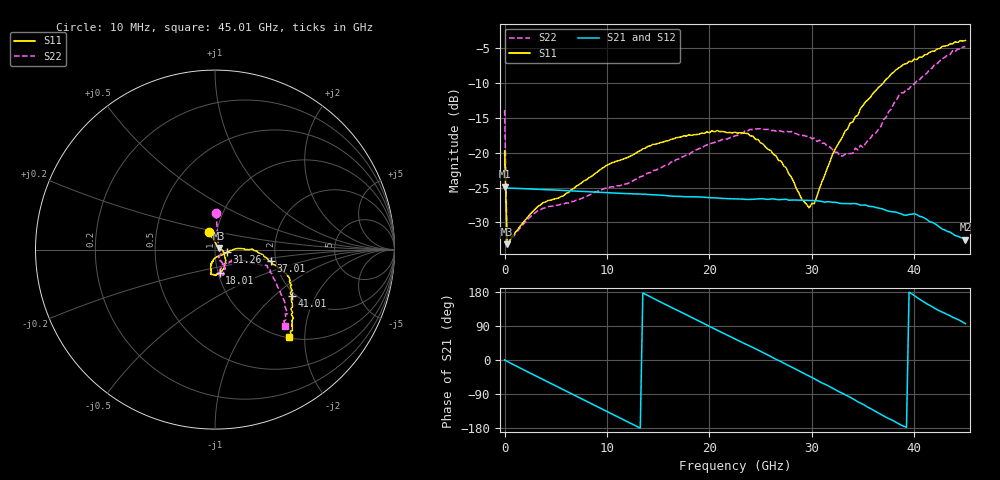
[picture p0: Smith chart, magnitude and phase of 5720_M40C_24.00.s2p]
! Device:  ADRF5720
! Description: 0.5dB LSB GaAs MMIC 6-bit Digital Attenuator
! Frequency:  0.000009 -  40 GHz
! Ports:
!	RF1	= Port 1
!	RF2	= Port 2
! Vdd:  3.3 Volt
! Vss:  -3.3 Volt
! Control:  0/3.3 Volt
! State:  24.00 dB attenuation
! Data:  The device was measured using G-S-G Probes on a matrix board.
!  Data was collected using an calibrated 4 port network analyzer.
!  The reference plane for this measurement is at the launchers.
! Note:  Analog Devices supplies this data as a sample of measured data
!  for this product.  Your particular data for this product may vary.
!  Data was taken at -40 degrees C.
!  Analog Devices reserves the right to change this data at anytime.
# GHZ S DB R 45.0
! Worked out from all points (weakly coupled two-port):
!   181 points, 10 MHz to 45.01 GHz, reference 45 ohm
!   highest |S21| = -24.90 dB at 10 MHz (marker M1); lowest = -32.5 dB at 45.01 GHz (marker M2)
!   lowest |S11| = -33.2 dB at 260 MHz (marker M3), VSWR 1.04, Z = 46.8 + j0.913 ohm
!   |S11| at or under -10 dB: start of sweep to 36.98 GHz
!   |S22| runs from -33.4 to -4.8 dB; largest |S21 - S12| = 0.00021
!   S11 on the Smith chart (normalised r, x): 10 MHz: 0.92, +0.18; 18.01 GHz: 1.02, -0.27; 31.26 GHz: 1.14, -0.03; 37.01 GHz: 1.88, -0.27; 41.01 GHz: 1.91, -1.33; 45.01 GHz: 1.02, -1.67
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0.01  -19.75 109.5  -24.90 0.3  -24.91 0.3  -13.88 88.3
0.26  -33.18 26.4  -25.08 -3.7  -25.10 -3.8  -33.42 22.4
3.26  -27.71 -4.6  -25.26 -44.8  -25.28 -44.8  -28.31 -29.3
7.76  -24.05 -32.4  -25.57 -105.5  -25.59 -105.5  -26.41 -62.0
15.26  -18.54 -67.0  -26.09 152.8  -26.11 152.7  -22.19 -62.0
18.01  -17.44 -78.9  -26.33 116.1  -26.36 116.0  -20.28 -60.7
22.76  -17.20 -99.0  -26.64 52.4  -26.67 52.3  -17.51 -69.1
24.26  -17.62 -100.1  -26.69 33.1  -26.71 33.0  -16.69 -71.2
26.01  -19.70 -103.6  -26.65 9.2  -26.68 9.1  -16.84 -75.3
27.51  -22.20 -101.9  -26.68 -11.8  -26.70 -11.9  -16.91 -78.7
29.01  -26.63 -90.5  -26.82 -32.0  -26.85 -32.1  -17.53 -81.4
29.76  -27.93 -63.5  -26.85 -42.6  -26.87 -42.8  -17.68 -81.5
30.26  -27.30 -42.5  -26.88 -49.5  -26.90 -49.6  -17.92 -80.0
31.26  -23.31 -11.6  -27.12 -63.5  -27.14 -63.6  -18.66 -75.1
32.76  -18.32 2.6  -27.27 -84.7  -27.29 -84.9  -20.46 -65.1
34.01  -15.60 -0.1  -27.30 -102.1  -27.32 -102.2  -20.09 -44.9
35.01  -13.22 -1.6  -27.53 -116.8  -27.56 -117.0  -19.24 -33.0
37.01  -9.95 -11.9  -28.12 -147.4  -28.14 -147.6  -15.27 -20.7
37.76  -8.70 -16.2  -28.46 -157.6  -28.48 -157.7  -13.75 -20.5
38.76  -7.56 -18.4  -28.78 -172.1  -28.80 -172.3  -11.41 -18.8
41.01  -5.97 -31.0  -29.38 152.3  -29.41 152.2  -8.82 -26.1
45.01  -3.89 -49.8  -32.50 95.9  -32.50 95.9  -4.78 -47.5
